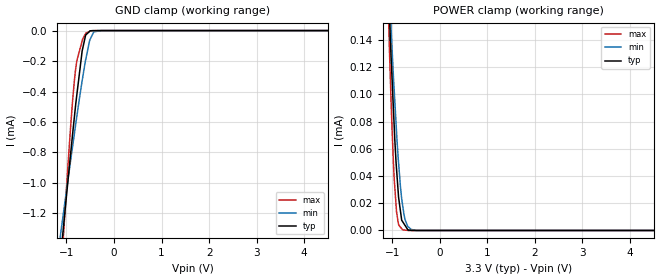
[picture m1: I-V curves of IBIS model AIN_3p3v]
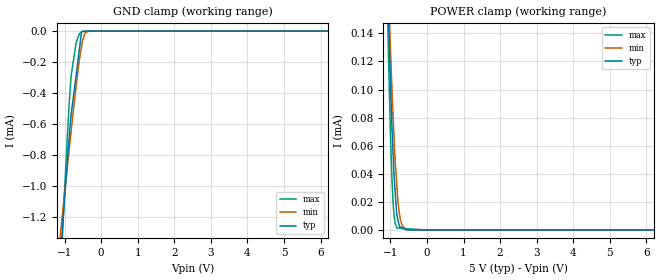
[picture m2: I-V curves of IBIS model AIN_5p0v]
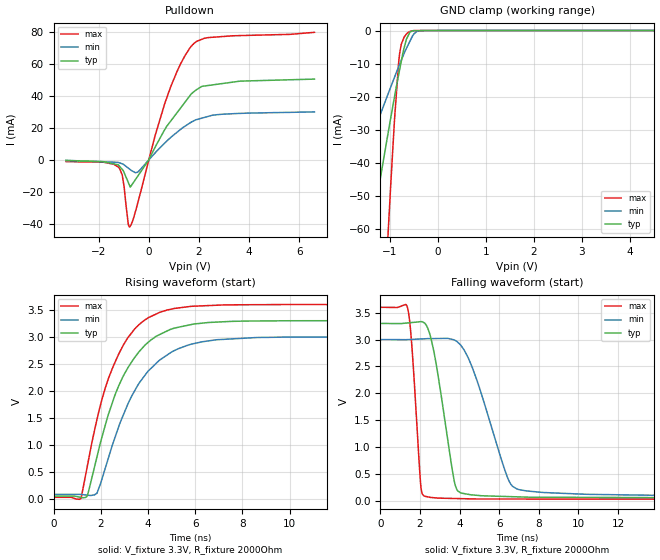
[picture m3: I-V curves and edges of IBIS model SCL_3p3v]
|Texas Instruments Incorporated
|4-wire resistive touch screen controller.
| Marketing part#   Voltage Range   Package-type   #pins
|ADS7828E/250   2.7 to 5.25V   TSSOP   16
|ADS7828E/250G4   2.7 to 5.25V   TSSOP   16
|ADS7828E/2K5   2.7 to 5.25V   TSSOP   16
|ADS7828E/2K5G4   2.7 to 5.25V   TSSOP   16
|ADS7828EB/250   2.7 to 5.25V   TSSOP   16
|ADS7828EB/250G4   2.7 to 5.25V   TSSOP   16
|ADS7828EB/2K5   2.7 to 5.25V   TSSOP   16
|ADS7828EB/2K5G4   2.7 to 5.25V   TSSOP   16
[IBIS Ver]   4.1
[File name]   ads7828.ibs
[File Rev]   1.0
[Date]   02/22/2011
[Source]   Texas Instruments Incorporated.
   Analog-eLab, HPA
   12500 TI Blvd
   Dallas, TX -75243
   For Support e-mail: elab_ibis@list.ti.com
[Notes]   Revision History:
   1.0: 02/03/2011
   - Initial version of the model
   - Initial Model generated from simulations.
   - Model names with a trailing _3p3v contains the model for
   3.3V (3.0V and 3.6V, +/- 10%). Model names with trailing _5p0v
   contains the model for 5V (4.75V and 5.25V, +/- 5%) operation.
   - Model not matched to measurements
   - Please ignore warnings related to non-monotonicity as they
   are from resutls of spice simulations.
[Disclaimer]
 This product is designed as an aid for customers of Texas Instruments.
 No warranties, either expressed or implied, with respect to this third
 party software (if any) or with respect to its fitness for any
 particular purpose is claimed by Texas Instruments or the author. The
 software (if any) is provided solely on an "as is" basis. The entire
 risk as to its quality and performance is with the customer
[Copyright] (C) Copyright 2011 Texas Instruments Incorporated.
   All rights reserved.
|   ADS7828
[Component]   ads7828
[Manufacturer] TI
[Package]   | 16 TSSOP  package
| variable   typ   min   max
R_pkg   0.04230125   0.02213   0.05369
L_pkg   2.32194nH   1.99467nH   3.0361nH
C_pkg   0.31027625pF   0.27895pF   0.39778pF
|-------------------------PIN------------------------------------------------
[Pin] signal_name  model_name  R_pin  L_pin C_pin
1   CH0   TERM   0.04574   3.0361nH   0.36595pF
2   CH1   TERM   0.0493   2.29713nH   0.29088pF
3   CH2   TERM   0.04301   2.07463nH   0.28195pF
4   CH3   TERM   0.04074   1.99687nH   0.27895pF
5   CH4   TERM   0.04113   2.01229nH   0.27999pF
6   CH5   TERM   0.0441   2.11766nH   0.28681pF
7   CH6   TERM   0.04911   2.29718nH   0.29455pF
8   CH7   TERM   0.03997   2.84895nH   0.35572pF
9   GND   GND   0.02213   2.60401nH   0.3869pF
10   REFIN_OUT   TERM   0.05369   2.45958nH   0.30451pF
11   COM   TERM   0.04656   2.20406nH   0.29493pF
12   A0   AIN   0.04186   2.03799nH   0.28368pF
13   A1   AIN   0.04067   1.99467nH   0.2803pF
14   SCL   SCL   0.04309   2.07723nH   0.2826pF
15   SDA   SDA   0.05208   2.39533nH   0.29892pF
16   VDD   POWER   0.02364   2.69736nH   0.39778pF
[Model Selector] AIN
AIN_3p3v   3.3V Address input
AIN_5p0v   5.0V Address input
[Model Selector] SCL
SCL_3p3v   3.3V SCL I/O
SCL_5p0v   5.0V SCL I/O
[Model Selector] SDA
SDA_3p3v   3.3V SDA I/O
SDA_5p0v   5.0V SDA I/O
|   TERM Model
[Model] TERM
Model_type Terminator
C_comp   0   0   0
| variable   typ   min   max
[Voltage Range]   3.3V   2.7V   5.25V
[POWER Clamp Reference]  3.3V   2.7V   5.25V
[GND Clamp Reference]   0.0V   0.0V   0.0V
|Operating Temperature
[Temperature Range]   27   85   -40
| Models and submodels in the file (7): AIN_3p3v (Input), AIN_5p0v (Input), SCL_3p3v (I/O_open_drain), SCL_5p0v (I/O_open_drain), SDA_3p3v (I/O_open_drain), SDA_5p0v (I/O_open_drain), TERM (Terminator)
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|   AIN_3p3v
[Model]   AIN_3p3v
Model_type   Input
Vinl = 0.99
Vinh = 2.31
|   typ   min   max
C_comp   1.850pF   1.839pF   1.863pF
[Voltage Range]   3.3   3   3.6
[Temperature Range]   27   85   -40
[Power Clamp Reference]   3.3   3   3.6
[GND Clamp Reference]   0   0   0
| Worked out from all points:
|   GND clamp passes 1 mA (typ) near -0.97 V on its own axis
|   POWER clamp passes 1 mA (typ) near -1.82 V on its own axis
[GND Clamp]
|   Voltage   I(typ)   I(min)   I(max)
-3.3V     -8.902mA   -6.56mA    -13.33mA
-1.157V   -1.602mA   -1.418mA   -1.828mA
-1.058V   -1.278mA   -1.188mA   -1.327mA
-909.5mV  -802.4uA   -849.2uA   -623.4uA
-812.7mV  -508.4uA   -632.4uA   -269.5uA
-782mV    -424.6uA   -565.2uA   -199.2uA
-669mV    -134.1uA   -329.3uA   -68.18uA
-595.8mV  -29.44uA   -192uA     -19.58uA
-499.1mV  -1.584uA   -56.22uA   -2.427uA
-424.1mV  -161.2nA   -8.151uA   -967.8nA
-264.1mV  -24.75nA   -66.25nA   0A
6.6V      0A         0A         0A
[POWER Clamp]
|   Voltage   I(typ)   I(min)   I(max)
-3.3V     2.806mA    2.316mA    3.762mA
-1.157V   254.3uA    255.7uA    259.7uA
-1.066V   164.4uA    181.5uA    141.7uA
-1.058V   158.1uA    175.8uA    132.7uA
-1.023V   126.8uA    147.3uA    93.87uA
-958.5mV  76.57uA    102.8uA    38uA
-909.5mV  45.33uA    72.47uA    13.9uA
-867.1mV  24.65uA    49.85uA    4.791uA
-782mV    6.512uA    18.73uA    478.1nA
-676.6mV  803.6nA    3.119uA    73.93nA
-509.9mV  4.581nA    60.72nA    0A
6.6V      0A         0A         0A
|   AIN_5p0v
[Model]   AIN_5p0v
Model_type   Input
Vinl = 1.5
Vinh = 3.5
|   typ   min   max
C_comp   1.849pF   1.838pF   1.862pF
[Voltage Range]   5   4.75   5.25
[Temperature Range]   27   85   -40
[Power Clamp Reference]   5   4.75   5.25
[GND Clamp Reference]   0   0   0
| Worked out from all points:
|   GND clamp passes 1 mA (typ) near -0.97 V on its own axis
[GND Clamp]
|   Voltage   I(typ)   I(min)   I(max)
-5V       -14.77mA   -10.7mA    -22.57mA
-1.126V   -1.5mA     -1.344mA   -1.667mA
-1.051V   -1.256mA   -1.171mA   -1.29mA
-902.6mV  -780.7uA   -832.8uA   -593.6uA
-820.1mV  -543uA     -648.3uA   -290.6uA
-682mV    -283.1uA   -355uA     -74.64uA
-601.3mV  -131.3uA   -201.7uA   -20.98uA
-534.1mV  -4.92uA    -99.24uA   -6.678uA
-511.6mV  -2.058uA   -66.65uA   -2.751uA
-434.4mV  -643.6nA   -11.03uA   -2.038uA
-341.5mV  -232.3nA   -473.4nA   -1.18uA
10V       0A         0A         0A
[POWER Clamp]
|   Voltage   I(typ)   I(min)   I(max)
-5V       4.92mA     4.029mA    6.652mA
-1.126V   224.8uA    228.9uA    217.3uA
-1.051V   153.8uA    169.5uA    124.1uA
-1.015V   119.3uA    141.1uA    86.04uA
-968.6mV  82.96uA    108.9uA    45.21uA
-919.1mV  50.9uA     78.12uA    17.5uA
-869.6mV  27.76uA    50.79uA    5.167uA
-820.1mV  11.11uA    31.26uA    1.349uA
-790.6mV  6.902uA    20.16uA    1.3uA
-723.5mV  1.957uA    7.103uA    1.187uA
-589.4mV  571.5nA    445.5nA    961.7nA
10V       0A         0A         0A
|   SCL_3p3v
[Model]   SCL_3p3v
Model_type   I/O_open_drain
Polarity   Non-Inverting
Enable   Active-High
Vinl = 0.99
Vinh = 2.31
Vmeas = 1.65
Vref = 1.65
Cref = 1pF
Rref = 50
|   typ   min   max
C_comp   0.523pF   0.451pF   0.561pF
[Voltage Range]   3.3   3   3.6
[Temperature Range]   27   85   -40
[Pullup Reference]   3.3   3   3.6
[Pulldown Reference]   0   0   0
[Power Clamp Reference]   3.3   3   3.6
[GND Clamp Reference]   0   0   0
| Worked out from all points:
|   slope of the pulldown table from 0 to 0.495 V, typ, clamps not added: 33.1 ohm
|   GND clamp passes 1 mA (typ) near -0.60 V on its own axis
|   falling waveform, V_fixture 3.3V, R_fixture 2000Ohm: 20-80 % time 811ps typ, 1.49ns min, 365ps max; typ from 3.3 V to 0.05 V
|   rising waveform, V_fixture 3.3V, R_fixture 2000Ohm: 20-80 % time 1.69ns typ, 1.87ns min, 1.52ns max; typ from 0.049 V to 3.3 V
[Pulldown]
|   Voltage   I(typ)   I(min)   I(max)
-3.3V     -421.7uA   -283.5uA   -1.075mA
-1.207V   -3.201mA   -1.634mA   -4.56mA
-1.059V   -5.95mA    -2.442mA   -9.342mA
-817.3mV  -14.06mA   -5.123mA   -40.06mA
-764.5mV  -16.01mA   -5.76mA    -42.01mA
-443.3mV  -10.25mA   -7.701mA   -27.15mA
669mV     19.79mA    11.01mA    36.67mA
1.249V    32.01mA    18.82mA    59.44mA
1.771V    42.23mA    24.2mA     72.33mA
2.118V    45.92mA    26.08mA    75.33mA
3.626V    49.15mA    29.04mA    77.61mA
6.6V      50.44mA    29.96mA    79.66mA
[GND Clamp]
|   Voltage   I(typ)   I(min)   I(max)
-3.3V     -229.6mA   -108.6mA   -718.4mA
-2.204V   -132.3mA   -64.83mA   -397.2mA
-2.013V   -115.5mA   -57.24mA   -341.2mA
-1.405V   -62.2mA    -33.27mA   -164.2mA
-1.059V   -32.59mA   -19.88mA   -66.46mA
-1.023V   -29.59mA   -18.52mA   -56.99mA
-905.6mV  -19.99mA   -14.12mA   -26.88mA
-799.7mV  -11.89mA   -10.25mA   -7.023mA
-656.2mV  -2.573mA   -5.357mA   -1.062mA
-555.1mV  -281.6uA   -2.377mA   -123.4uA
-291.9mV  -35.53uA   -1.967uA   0A
6.6V      0A         0A         0A
[POWER Clamp]
|   Voltage   I(typ)   I(min)   I(max)
-3.3V     0A         0A         0A
0V        0A         0A         0A
6.6V      0A         0A         0A
[Ramp]
R_load = 2000
|   typ   min   max
dV/dt_r   1.95079/1.69655e-009   1.75119/1.85441e-009   2.14396/1.51787e-009
dV/dt_f   1.95006/8.10926e-010   1.74662/1.48898e-009   2.14394/3.64926e-010
[Falling Waveform]
V_fixture = 3.3V
V_fixture_min = 3V
V_fixture_max = 3.6V
R_fixture = 2000Ohm
C_fixture = 0F
|   Time   V(typ)   V(min)   V(max)
0s        3.3V       3V         3.6V
1.371ns   3.309V     2.999V     3.594V
1.59ns    3.317V     3.003V     2.871V
2.028ns   3.333V     3.011V     327mV
2.208ns   3.312V     3.014V     89.28mV
2.721ns   2.738V     3.019V     55.82mV
3.734ns   358.7mV    2.993V     42.31mV
4.046ns   148.7mV    2.901V     39.71mV
6.903ns   73.26mV    218.3mV    32.51mV
21.04ns   49.91mV    88.97mV    26.77mV
[Rising Waveform]
V_fixture = 3.3V
V_fixture_min = 3V
V_fixture_max = 3.6V
R_fixture = 2000Ohm
C_fixture = 0F
|   Time   V(typ)   V(min)   V(max)
0s        48.68mV    81.33mV    26.73mV
1.155ns   26.96mV    80.78mV    1.217mV
1.441ns   69.15mV    66.39mV    626.9mV
1.837ns   771.3mV    100.2mV    1.463V
2.344ns   1.59V      785.1mV    2.252V
2.954ns   2.274V     1.551V     2.846V
3.643ns   2.735V     2.154V     3.235V
4.522ns   3.048V     2.578V     3.459V
6.903ns   3.274V     2.947V     3.586V
21.04ns   3.3V       3V         3.6V
